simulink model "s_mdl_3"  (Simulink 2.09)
settings: Solver=ode15s  StartTime=0.0  StopTime=1000  RelTol=1e-3  AbsTol=1e-6

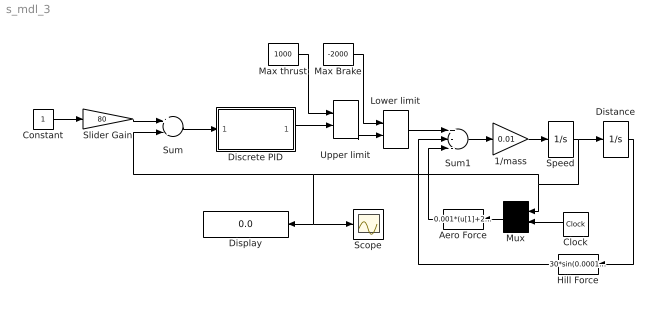
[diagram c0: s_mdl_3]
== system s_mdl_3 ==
  1/mass : Gain  Gain=0.01
  Aero Force : Fcn  Orientation=left  Expr=0.001*(u[1]+20*sin(0.01*u[2]))^2
  Clock : Clock
  Constant : Constant  Value=1
  Discrete PID : Subsystem  mask(Discrete PID Controller){Kp=50, Ki=0.75, Kd=75, L_upper=100, L_lower=-100, T_samp=0.5}
      mask prompts: Kp "Proportional gain:"; Ki "Integral gain:"; Kd "Derivative gain:"; L_upper "Upper saturation limit:"; L_lower "Lower saturation limit:"; T_samp "Sample period"
  Display : Display
  Distance : Integrator  ExternalReset=none  InitialConditionSource=internal  InitialCondition=0  LimitOutput=off  UpperSaturationLimit=inf  LowerSaturationLimit=-inf  ShowSaturationPort=off  ShowStatePort=off  AbsoluteTolerance=auto
  Hill Force : Fcn  Orientation=left  Expr=30*sin(0.0001*u[1])
  Lower limit : MinMax  Function=max  Inputs=2
  Max Brake : Constant  Value=-2000
  Max thrust : Constant  Value=1000
  Mux : Mux  Orientation=left  Inputs=2
  Scope : Scope
  Slider Gain : Gain  LoadFcn=slideg Load  Gain=80  mask(Slider Gain){}
  Speed : Integrator  ExternalReset=none  InitialConditionSource=internal  InitialCondition=0  LimitOutput=off  UpperSaturationLimit=inf  LowerSaturationLimit=-inf  ShowSaturationPort=off  ShowStatePort=off  AbsoluteTolerance=auto
  Sum : Sum  Inputs=+-
  Sum1 : Sum  Inputs=+--
  Upper limit : MinMax  Function=min  Inputs=2
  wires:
  Discrete PID/1(Control) -> Upper limit/2
  Sum/1 -> Discrete PID/1(Error in)
  Speed/1 -> Distance/1, Mux/1, Sum/2, Scope/1, Display/1
  Clock/1 -> Mux/2
  Lower limit/1 -> Sum1/1
  Max Brake/1 -> Lower limit/1
  Max thrust/1 -> Upper limit/1
  Upper limit/1 -> Lower limit/2
  1/mass/1 -> Speed/1
  Sum1/1 -> 1/mass/1
  Distance/1 -> Hill Force/1
  Hill Force/1 -> Sum1/2
  Aero Force/1 -> Sum1/3
  Mux/1 -> Aero Force/1
  Constant/1 -> Slider Gain/1
  Slider Gain/1 -> Sum/1

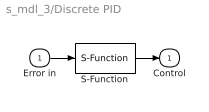
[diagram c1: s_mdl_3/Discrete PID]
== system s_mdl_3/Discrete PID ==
  Error in : Inport  Port=1  PortWidth=-1  SampleTime=-1
  S-Function : S-Function  FunctionName=s_xmp3  Parameters=Kp, Ki, Kd, L_upper, L_lower, T_samp
  Control : Outport  Port=1  InitialOutput=0
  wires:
  S-Function/1 -> Control/1
  Error in/1 -> S-Function/1
